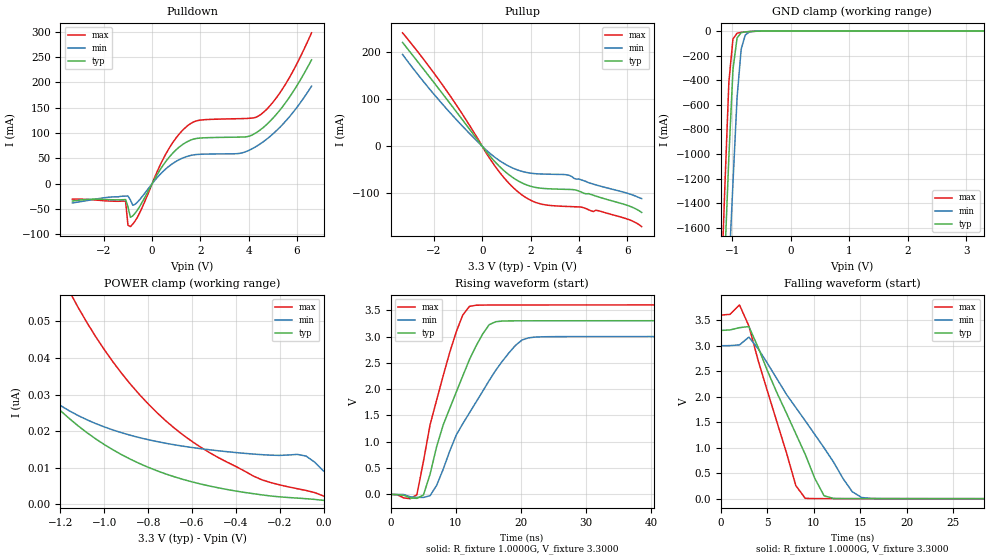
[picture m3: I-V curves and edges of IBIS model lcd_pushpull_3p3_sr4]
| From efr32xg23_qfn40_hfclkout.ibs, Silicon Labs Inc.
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|   Model lcd_pushpull_3p3_sr4
[Model]  lcd_pushpull_3p3_sr4
Model_type 3-state
Polarity   Non-Inverting
Enable   Active-High
C_comp   1.6300pF   1.4000pF   2.7000pF
[Temperature Range]   25.0000   0.1250k   -40.0000
[Pullup Reference]   3.3000V   3.0000V   3.6000V
[Pulldown Reference]   0.0V   0.0V   0.0V
[POWER Clamp Reference]   3.3000V   3.0000V   3.6000V
[GND Clamp Reference]   0.0V   0.0V   0.0V
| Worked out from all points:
|   slope of the pulldown table from 0 to 0.495 V, typ, clamps not added: 12.6 ohm
|   slope of the pullup table from 0 to 0.495 V, typ, clamps not added: 15.9 ohm
|   GND clamp passes 1 mA (typ) near -0.56 V on its own axis
|   rising waveform, R_fixture 1.0000G, V_fixture 3.3000: 20-80 % time 5.82ns typ, 7.96ns min, 4.37ns max; typ from 0 V to 3.3 V
|   falling waveform, R_fixture 1.0000G, V_fixture 3.3000: 20-80 % time 4.81ns typ, 6.62ns min, 3.58ns max; typ from 3.3 V to 0 V
[Pulldown]
|Voltage   I(typ)   I(min)   I(max)
-3.3V     -34.2mA    -37.99mA   -30.45mA
-1.1V     -31.33mA   -24.53mA   -34.17mA
-1V       -45.32mA   -24.25mA   -81.91mA
-900mV    -66.33mA   -32.01mA   -84.65mA
-700mV    -57.95mA   -40.56mA   -73.32mA
500mV     39.57mA    26.37mA    52.76mA
1.2V      75.23mA    49.28mA    102.4mA
1.9V      89.73mA    57.85mA    124.8mA
3.6V      92mA       59.71mA    128.4mA
4.5V      107.1mA    79.43mA    136.7mA
5.5V      158.4mA    122.1mA    194.8mA
6.6V      244.5mA    192.6mA    297.9mA
[Pullup]
|Voltage   I(typ)   I(min)   I(max)
-3.3V     221.2mA    195.6mA    241.7mA
-1.7V     115.8mA    92.91mA    134.7mA
-200mV    13.9mA     10.19mA    17.6mA
200mV     -13.41mA   -9.668mA   -17.24mA
700mV     -42.19mA   -29.99mA   -54.16mA
1.5V      -74.1mA    -51.07mA   -97.84mA
1.9V      -83.4mA    -56.39mA   -112mA
2.4V      -89.1mA    -58.9mA    -122.5mA
3.6V      -91.86mA   -61.88mA   -128.3mA
4.9V      -109.2mA   -84.97mA   -138.5mA
6.1V      -127.5mA   -101.5mA   -156.7mA
6.6V      -140.8mA   -111.3mA   -171mA
[GND_clamp]
|Voltage   I(typ)   I(min)   I(max)
-3.3V     -27.87A    -25.05A    -30.64A
-1.2V     -2.686A    -3.389A    -2.22A
-1.13V    -1.852A    -2.669A    -1.282A
-1.06V    -1.021A    -1.951A    -413.8mA
-990mV    -311.8mA   -1.235A    -64.72mA
-920mV    -56.25mA   -542.5mA   -17.8mA
-850mV    -13.45mA   -148.5mA   -11.08mA
-780mV    -6.591mA   -32.68mA   -7.457mA
-710mV    -4.029mA   -8.323mA   -4.574mA
-360mV    -18.91uA   -70.05uA   -6.844uA
3.3V      1.07nA     13.64nA    781.9pA
[POWER_clamp]
|Voltage   I(typ)   I(min)   I(max)
-3.28V    727.8nA    32.99uA    1.086uA
-1.6V     57.64nA    55.61nA    128.6nA
-1.56V    53.42nA    50.92nA    120.3nA
-1.4V     38.98nA    37.13nA    91.2nA
-1.16V    23.46nA    25.56nA    58.31nA
-1.12V    21.47nA    24.28nA    53.91nA
-880mV    12.29nA    18.85nA    32.79nA
-640mV    6.783nA    15.87nA    18.92nA
-320mV    2.894nA    13.73nA    7.713nA
-120mV    1.684nA    13.64nA    4.257nA
-80mV     1.52nA     13.19nA    3.779nA
0V        1.07nA     9.091nA    2.25nA
[Ramp]
| variable   typ   min   max
dV/dt_r  1.9770/5.9951n   1.7962/8.2862n   2.1574/4.4586n
dV/dt_f  1.9778/4.8894n   1.7971/6.7846n   2.1582/3.6196n
R_load = 10.0000k
[Rising Waveform]
R_fixture= 1.0000G
V_fixture= 3.3000
V_fixture_min= 3.0000
V_fixture_max= 3.6000
|time   V(typ)   V(min)   V(max)
0s        3.773uV    9.216uV    2.015uV
4.04ns    -75.1mV    -55.83mV   -6.488mV
5.051ns   -11.4mV    -58.47mV   629.8mV
6.061ns   380.1mV    -24.92mV   1.319V
8.081ns   1.319V     477.3mV    2.255V
10.1ns    1.949V     1.131V     3.095V
12.12ns   2.564V     1.55V      3.573V
15.15ns   3.225V     2.164V     3.598V
21.21ns   3.298V     2.975V     3.599V
100ns     3.3V       3V         3.6V
[Falling Waveform]
R_fixture= 1.0000G
V_fixture= 3.3000
V_fixture_min= 3.0000
V_fixture_max= 3.6000
|time   V(typ)   V(min)   V(max)
0s        3.3V       3V         3.6V
1.01ns    3.31V      3.002V     3.616V
2.02ns    3.354V     3.016V     3.8V
3.03ns    3.375V     3.169V     3.387V
8.081ns   1.272V     1.786V     254.8mV
9.091ns   868.8mV    1.528V     6.911mV
11.11ns   57.75mV    997.9mV    1.028mV
14.14ns   1.385mV    137.9mV    563.6uV
16.16ns   886.7uV    5.629mV    441.8uV
100ns     3.911uV    9.411uV    2.098uV
